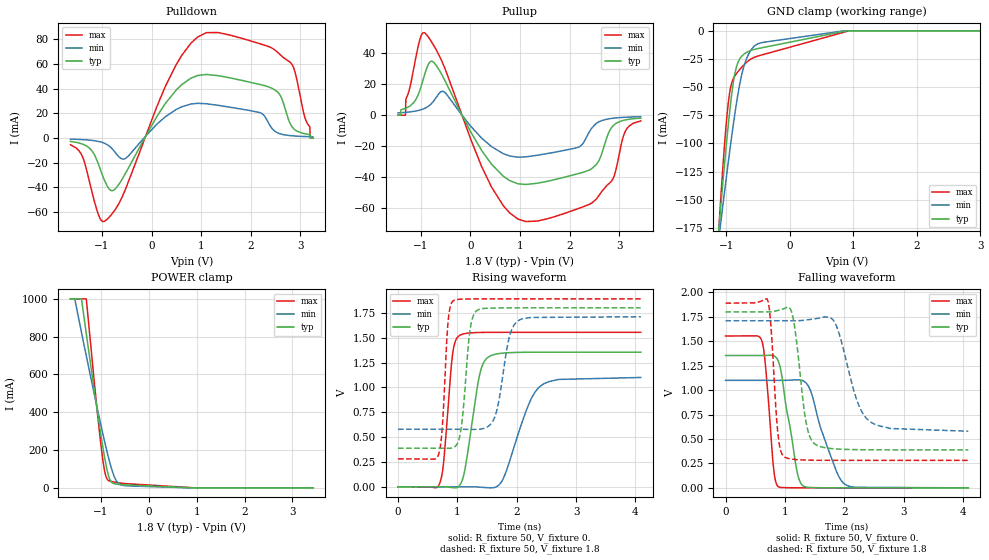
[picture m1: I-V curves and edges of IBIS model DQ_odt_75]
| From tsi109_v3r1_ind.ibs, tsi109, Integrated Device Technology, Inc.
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|   MODEL DQ_odt_75
[Model]   DQ_odt_75
Model_type  I/O
Polarity   Non-Inverting
Enable   Active-Low
|   typ   min   max
|C_comp_off 3.363p 3.358p 3.318p
|C_comp_on 3.698p 3.56p 3.948p
C_comp 3.53p 3.459p 3.633p
Cref  =   20pF
Vmeas =   0.9v
Vinl  =   0.650v
Vinh  =   1.150v
[Model Spec]
[Temperature Range]   25   125   -40
[Voltage Range] 1.8 1.71 1.89
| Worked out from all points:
|   slope of the pulldown table from 0 to 0.27 V, typ, clamps not added: 15.3 ohm
|   slope of the pullup table from 0 to 0.27 V, typ, clamps not added: 18.8 ohm
|   rising waveform, R_fixture 50, V_fixture 0.: 20-80 % time 205ps typ, 380ps min, 124ps max; typ from 0 V to 1.35 V
|   rising waveform, R_fixture 50, V_fixture 1.8: 20-80 % time 121ps typ, 188ps min, 85.6ps max; typ from 0.389 V to 1.8 V
|   falling waveform, R_fixture 50, V_fixture 0.: 20-80 % time 211ps typ, 348ps min, 119ps max; typ from 1.35 V to 0 V
|   falling waveform, R_fixture 50, V_fixture 1.8: 20-80 % time 164ps typ, 316ps min, 100ps max; typ from 1.8 V to 0.389 V
[Pulldown]
-1.636V   -2.749mA   -869.2uA   -5.387mA
-1.394V   -4.913mA   -1.288mA   -15.17mA
-1.215V   -9.752mA   -1.87mA    -41.58mA
-1.037V   -25.03mA   -3.084mA   -65.39mA
-898.6mV  -38.74mA   -5.29mA    -65.92mA
-552.1mV  -30.44mA   -16.98mA   -43.89mA
492.4mV   38.76mA    23.09mA    59.27mA
1.106V    51.56mA    27.79mA    85.47mA
2.195V    43.31mA    20.48mA    76.3mA
2.487V    38.92mA    5.461mA    71.35mA
2.809V    10.58mA    1.904mA    60.81mA
3.26V     0A         0A         0A
[Pullup]
-1.46V    0A         1.493mA    0A
-1.311V   4.439mA    1.848mA    0A
-1.044V   13.88mA    3.125mA    45.65mA
-915.1mV  26.96mA    4.523mA    53mA
-533.9mV  23.65mA    15.18mA    31.79mA
426.4mV   -31.56mA   -20.23mA   -46.29mA
1.119V    -44.65mA   -26.83mA   -68.55mA
2.204V    -37.38mA   -20.25mA   -59.84mA
2.535V    -31.95mA   -5.371mA   -54.19mA
2.877V    -6.877mA   -1.927mA   -40.86mA
3.119V    -3.056mA   -1.316mA   -10.73mA
3.436V    -1.832mA   -944.9uA   -3.621mA
[GND Clamp]
-1.636V   -544.5mA   -441.7mA   -699.3mA
-1.118V   -178.8mA   -186.7mA   -179.7mA
-1.093V   -162.3mA   -174.9mA   -157.4mA
-998.9mV  -102.8mA   -131.4mA   -83.18mA
-959.1mV  -80.05mA   -113.8mA   -61.12mA
-924.2mV  -62.17mA   -98.82mA   -48.97mA
-844.6mV  -33.7mA    -67.13mA   -38.63mA
-735mV    -21.49mA   -34.58mA   -31.11mA
-640.4mV  -18.12mA   -20.15mA   -26.22mA
-521mV    -16.02mA   -12.1mA    -22.8mA
930.2mV   0A         0A         0A
3.26V     0A         0A         0A
[Power Clamp]
-1.636V   1A         1A         1A
-1.546V   1A         997.4mA    1A
-1.407V   998.4mA    824mA      1A
-1.307V   818.5mA    700.4mA    1A
-1.078V   409.6mA    422.6mA    408.4mA
-998mV    276.2mA    329.6mA    223.6mA
-918.2mV  154.6mA    240.1mA    83.97mA
-848.4mV  71mA       166.8mA    40.12mA
-783.6mV  31.4mA     106.1mA    33.79mA
-693.8mV  20.28mA    44.56mA    29.34mA
-514.3mV  16.05mA    11.88mA    23.15mA
3.436V    0A         0A         0A
[Ramp]
dV/dt_r .812/205.375p .66/380.602p .932/123.936p
dV/dt_f .847/163.938p .679/315.888p .965/99.968p
[Rising Waveform]
R_fixture = 50
V_fixture = 0.
0s        0V         0V         0V
700ps     244.5uV    -2.152uV   31.55mV
770ps     49.9uV     875.3nV    255.6mV
920ps     -8.207mV   73.82uV    1.334V
1.04ns    16.71mV    185.6uV    1.523V
1.37ns    1.113V     -2.911mV   1.552V
1.51ns    1.299V     -9.011mV   1.553V
1.77ns    1.345V     78.26mV    1.554V
2.43ns    1.354V     1.026V     1.554V
4.09ns    1.354V     1.1V       1.554V
[Rising Waveform]
R_fixture = 50
V_fixture = 1.8
V_fixture_min = 1.71
V_fixture_max = 1.89
0s        388.5mV    578.6mV    281mV
680ps     388.4mV    578.7mV    318.7mV
740ps     388mV      578.7mV    550.7mV
850ps     387.5mV    578.7mV    1.696V
940ps     397.2mV    578.7mV    1.875V
1.05ns    535.1mV    578.4mV    1.886V
1.33ns    1.773V     577.6mV    1.89V
1.63ns    1.798V     701.1mV    1.89V
2.03ns    1.8V       1.672V     1.89V
4.09ns    1.8V       1.71V      1.89V
[Falling Waveform]
R_fixture = 50
V_fixture = 0.
0s        1.354V     1.1V       1.554V
620ps     1.354V     1.1V       1.491V
680ps     1.355V     1.1V       1.208V
820ps     1.349V     1.1V       145.9mV
900ps     1.278V     1.1V       8.41mV
1.2ns     183.3mV    1.105V     710uV
1.31ns    19.37mV    1.094V     400.2uV
1.86ns    480.7uV    183.1mV    21.03uV
2.02ns    258.4uV    33.45mV    9.172uV
4.09ns    0V         23.14uV    0V
[Falling Waveform]
R_fixture = 50
V_fixture = 1.8
V_fixture_min = 1.71
V_fixture_max = 1.89
0s        1.8V       1.71V      1.89V
720ps     1.8V       1.71V      1.903V
880ps     1.815V     1.71V      568.6mV
1ns       1.837V     1.71V      313.4mV
1.13ns    1.762V     1.71V      293.2mV
1.35ns    695.3mV    1.717V     284.2mV
1.51ns    446.5mV    1.73V      282.3mV
1.84ns    399.2mV    1.694V     281.2mV
2.42ns    389.6mV    685.4mV    281mV
4.09ns    388.5mV    579.6mV    281mV
